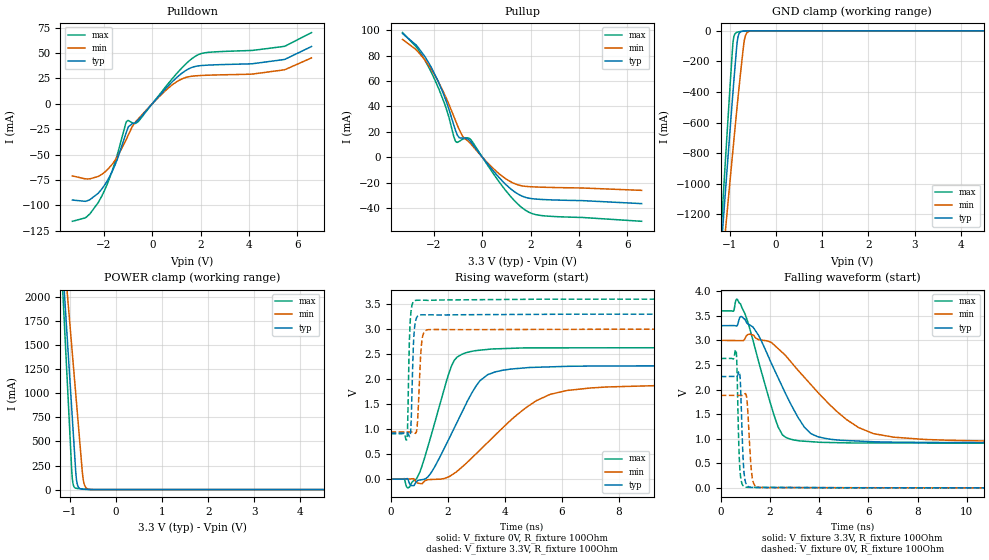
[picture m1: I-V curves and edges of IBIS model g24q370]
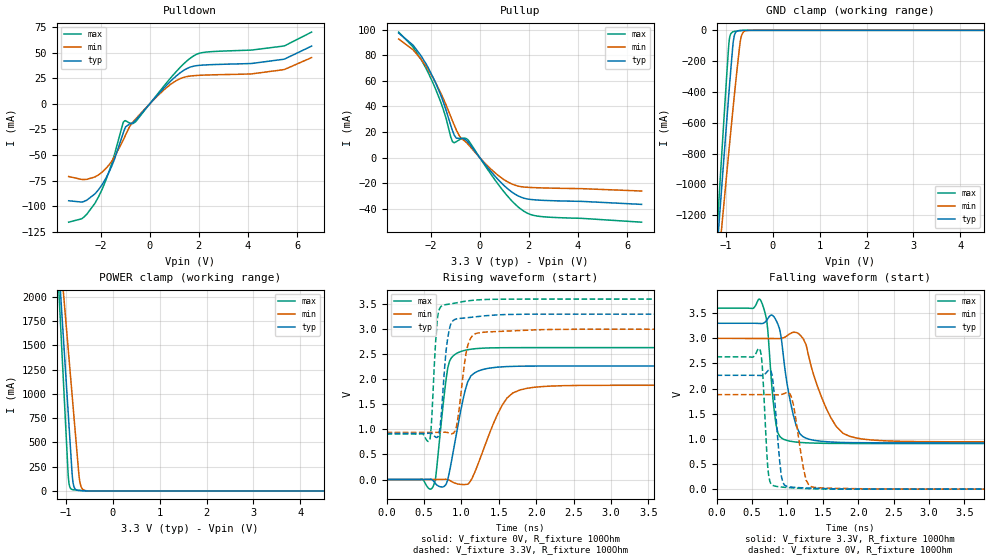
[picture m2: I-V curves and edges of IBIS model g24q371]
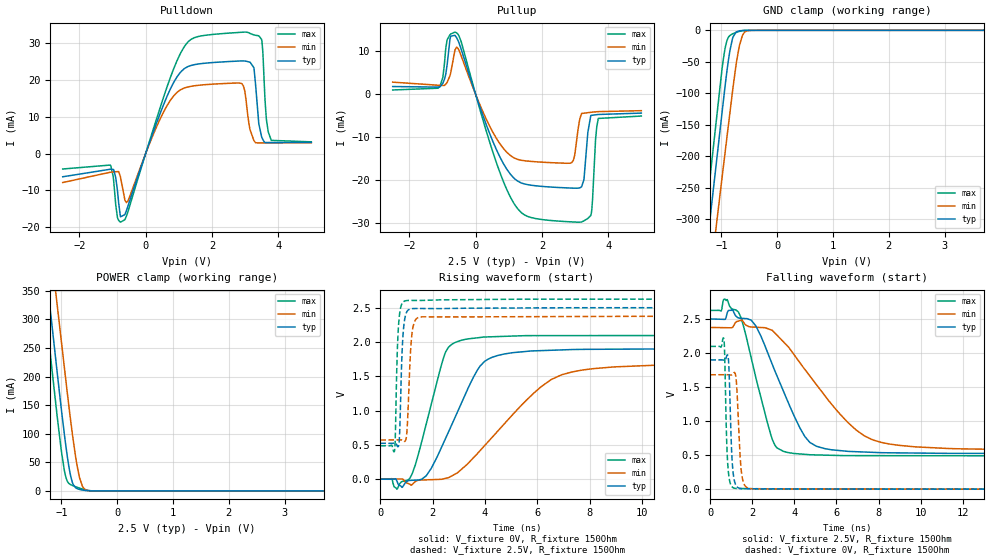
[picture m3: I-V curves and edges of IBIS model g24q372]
| Texas Instruments Incorporated
| Single Port 10/100 Mbps Eth Phys Layer Transceiver w/ Fiber Support
| Marketing part#   Voltage Range   Package-type   #pins/pkg drawing
| DP83620   2.375V - 3.6V   LLP   48-pin LLP
[IBIS Ver]   4.1
[Comment char]  |_char
[File name]   dp83620.ibs
[File Rev]   1.2
[Date]   11/01/2016
[Source]   Model built from spectre simulations at:
   Texas Instruments Incorporated.
   Analog-eLab, HPA
   12500 TI Blvd
   Dallas, TX -75243
   For Support e-mail: elab_ibis@list.ti.com
[Notes]   Revision History
   Rev 1.2: 11/1/2016
   - Update g24q370, g27q371 from DP83630
   Rev 1.1: 6/15/2016
   - New model for g24q37x buffer I/O at 2.5V operation.
   Rev 1.0: 05/2/2011
   -Pulldown & pullup non-monotonic for g24q37x modes reflect buffer behavior
   -osc25x1 POWER Clamp model stops at VCC. GND clamp shows 0 current at 0V.
   - C_comp although listed in numerical order of value are obtained from varying PVT conditions.
   For PVT conditions for each specific value, refer to the buffer description under respective [Model].
   IBIS model user is responsible for using appropriate C_comp to simulate for Signal Integrity.
[Disclaimer]  This model is designed as an aid for customers of Texas Instruments
 TI and its licensors and suppliers make no warranties, either expressed
 or implied, with respect to this  model, including the warranties of
 merchantability or fitness for a particular purpose.
 The model is provided solely on an "as is" basis. The entire risk as to
 its quality and performance is with the customer.
[Copyright] (C)Copyright 2016 Texas Instruments Incorporated.
   All rights reserved.
[Component]   DP83620
[Manufacturer]  Texas Instruments
[Package]
|   typ   min   max
R_pkg   0.359   0.180   0.442
L_pkg   2.373n   1.687n   2.945n
C_pkg   0.123p   0.108p   0.150p
[Pin]   signal_name   model_name   R_pin   L_pin   C_pin
1   TX_CLK   g24q37x   0.42936   2.873n   0.148196p
2   TX_EN   g24q37x   0.40013   2.628n   0.124306p
3   TXD_0   g24q37x   0.37267   2.418n   0.119907p
4   TXD_1   g24q37x   0.35187   2.266n   0.118634p
5   TXD_2   g24q37x   0.33473   2.147n   0.117883p
6   TXD_3   g24q37x   0.32586   2.085n   0.119334p
7   PWRDOWN/INTN   g24q37x   0.32558   2.084n   0.119406p
8   TCK   g24q37x   0.33356   2.137n   0.118268p
9   TDO   g24q37x   0.34873   2.244n   0.118339p
10   TMS   g24q37x   0.36988   2.399n   0.119828p
11   TRST#   g24q37x   0.39607   2.598n   0.123672p
12   TDI   g24q37x   0.42596   2.846n   0.146171p
13   RD-   NC   0.42552   2.846n   0.138036p
14   RD+   NC   0.39994   2.586n   0.114697p
15   CD_VSS   GND   0.21019   1.982n   0.12691p
16   TD-   NC   0.35238   2.219n   0.10829p
17   TD+   NC   0.33431   2.112n   0.109207p
18   ANAVSS   GND   0.18023   1.687n   0.130115p
19   ANA33VDD   POWER   0.32768   2.094n   0.114926p
20   VREF   NC   0.33377   2.159n   0.121083p
21   CLK_OUT_EN   g24q37x   0.34083   2.203n   0.118534p
22   PCF_EN   g24q37x   0.36206   2.35n   0.116057p
23   RESERVED   g24q37x   0.38591   2.551n   0.124689p
24   CLK_OUT   g24q37x   0.43535   2.929n   0.144582p
25   RESERVED   g24q37x   0.44243   2.945n   0.143157p
26   LED_ACT   g24q37x   0.40924   2.689n   0.124605p
27   LED_SPEED   g24q37x   0.38041   2.477n   0.121061p
28   LED_LINK   g24q37x   0.35858   2.311n   0.119803p
29   RESET_N   g24q37x   0.34101   2.179n   0.117093p
30   MDIO   g24q37x   0.32959   2.091n   0.115554p
31   MDC   g24q37x   0.32689   2.082n   0.117569p
32   IO_VDD   POWER   0.33388   2.126n   0.116848p
33   X2   osc25x2   0.35262   2.24n   0.115121p
34   X1   osc25x1   0.37844   2.403n   0.116058p
35   IO_CORE_VSS   GND   0.21929   2.112n   0.150154p
36   RESERVED   g24q37x   0.41951   2.799n   0.146508p
37   RESERVED   g24q37x   0.42645   2.861n   0.136214p
38   RX_CLK   g24q37x   0.40341   2.667n   0.120159p
39   RX_DV   g24q37x   0.37560   2.446n   0.114535p
40   CRS/CRS_DV   g24q37x   0.35301   2.276n   0.112899p
41   RX_ER   g24q37x   0.33596   2.154n   0.111927p
42   COL   g24q37x   0.32709   2.092n   0.111756p
43   RXD_3   g24q37x   0.32713   2.092n   0.11131p
44   RXD_2   g24q37x   0.33667   2.162n   0.112238p
45   RXD_1   g24q37x   0.35414   2.288n   0.113403p
46   RXD_0   g24q37x   0.37605   2.462n   0.117967p
47   IO_VSS   GND   0.39618   2.621n   0.122466p
48   IO_VDD   POWER   0.42506   2.862n   0.142308p
[Diff_pin]   inv_pin   vdiff   tdelay_typ   tdelay_min   tdelay_max
| The '+' pin is Diff_pin and the '-' pin is the inv_pin
14   13   0.100   0 0 0
17   16   0.100   0 0 0
[Model Selector]   g24q37x
g24q370   mode: SS = VSS, VDD = 3.3
g24q371   mode: SS = VDD, VDD = 3.3
g24q372   mode: SS = VSS, VDD = 2.5
g24q373   mode: SS = VDD, VDD = 2.5
| Models and submodels in the file (6): g24q370 (I/O), g24q371 (I/O), g24q372 (I/O), g24q373 (I/O), osc25x1 (Input), osc25x2 (Output)
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|   Model g24q370
[Model]   g24q370
Model_type   I/O
Polarity   Non-Inverting
Enable   Active-Low
Vinl = 0.8
Vinh = 2.0
Vmeas = 1.5
|   typ   min   max
C_comp   1.0640pF   1.0620pF   1.0670pF
[Voltage Range]   3.3   3   3.6
[Temperature Range]   25   125   -40
[Pullup Reference]   3.3   3   3.6
[Pulldown Reference]   0   0   0
[Power Clamp Reference]   3.3   3   3.6
[GND Clamp Reference]   0   0   0
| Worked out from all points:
|   slope of the pulldown table from 0 to 0.495 V, typ, clamps not added: 37.3 ohm
|   slope of the pullup table from 0 to 0.495 V, typ, clamps not added: 42.1 ohm
|   GND clamp passes 1 mA (typ) near -0.69 V on its own axis
|   POWER clamp passes 1 mA (typ) near -0.59 V on its own axis
|   falling waveform, V_fixture 3.3V, R_fixture 100Ohm: 20-80 % time 1.39ns typ, 2.41ns min, 911ps max; typ from 3.3 V to 0.919 V
|   rising waveform, V_fixture 0V, R_fixture 100Ohm: 20-80 % time 1.21ns typ, 2.18ns min, 795ps max; typ from 0 V to 2.27 V
|   rising waveform, V_fixture 3.3V, R_fixture 100Ohm: 20-80 % time 79.2ps typ, 104ps min, 68.6ps max; typ from 0.919 V to 3.3 V
|   falling waveform, V_fixture 0V, R_fixture 100Ohm: 20-80 % time 102ps typ, 134ps min, 86.2ps max; typ from 2.27 V to 0 V
[Pulldown]
|   Voltage   I(typ)   I(min)   I(max)
-3.3V     -94.78mA   -71.06mA   -115.7mA
-2.676V   -95.44mA   -74.02mA   -110.7mA
-2.092V   -84.17mA   -69.57mA   -91.23mA
-1.558V   -61.46mA   -56.42mA   -59.08mA
-1.073V   -28.13mA   -35.11mA   -17.82mA
-983.4mV  -22.58mA   -30.44mA   -16.52mA
-577.5mV  -16.03mA   -14.92mA   -17.52mA
838.2mV   21.93mA    18.83mA    24.99mA
1.62V     35.69mA    27.12mA    44.11mA
2.224V    38.02mA    28.13mA    50.44mA
5.452V    43.63mA    33.46mA    56.55mA
6.59V     56.49mA    45.27mA    70.2mA
[GND Clamp]
|   Voltage   I(typ)   I(min)   I(max)
-3.3V     -10.39A    -8.782A    -12.22A
-1.191V   -1.434A    -1.613A    -1.311A
-1.122V   -1.151A    -1.385A    -967.2mA
-1.102V   -1.07A     -1.32A     -869.6mA
-1.043V   -830.1mA   -1.127A    -579.2mA
-933.9mV  -400mA     -776mA     -77.86mA
-854.7mV  -108.3mA   -528mA     -9.646mA
-805.2mV  -20.45mA   -378.7mA   -6.059mA
-696.3mV  -1.135mA   -78.24mA   -2.129mA
-646.8mV  -417.3uA   -19.97mA   -1.017mA
-577.5mV  -93.99uA   -2.797mA   -240.5uA
6.59V     0A         0A         0A
[Pullup]
|   Voltage   I(typ)   I(min)   I(max)
-3.3V     97.33mA    92.68mA    98.1mA
-2.686V   87.17mA    83.6mA     85.57mA
-2.102V   70.37mA    68.84mA    66.51mA
-1.518V   45.28mA    47.6mA     39.67mA
-1.102V   20.69mA    28.41mA    12.28mA
-953.7mV  15.22mA    21.61mA    12.45mA
-825mV    15.02mA    16.78mA    13.99mA
-468.6mV  11.9mA     10.27mA    13.6mA
699.6mV   -16.19mA   -13.13mA   -19.54mA
1.67V     -30.88mA   -22.7mA    -40.23mA
2.501V    -33.35mA   -23.67mA   -46.09mA
6.59V     -36.58mA   -26.14mA   -50.5mA
[POWER Clamp]
|   Voltage   I(typ)   I(min)   I(max)
-3.3V     19.11A     15.19A     23.53A
-1.241V   2.989A     3.111A     2.924A
-963.6mV  899.3mA    1.533A     275.2mA
-953.7mV  824.7mA    1.477A     183.3mA
-933.9mV  675.5mA    1.365A     79.06mA
-874.5mV  227.9mA    1.027A     16.17mA
-854.7mV  111.6mA    914.3mA    13.23mA
-825mV    39.61mA    745.4mA    11.03mA
-716.1mV  3.952mA    138.9mA    6.502mA
-676.5mV  2.669mA    45.08mA    5.111mA
-597.3mV  1.12mA     4.928mA    2.691mA
6.59V     0A         0A         0A
[Ramp]
R_load = 100
|   typ   min   max
dV/dt_r   1.35904/1.20591e-09   1.12844/2.184e-09   1.57884/7.94904e-10
dV/dt_f   1.42833/1.38701e-09   1.2344/2.40837e-09   1.61561/9.11184e-10
[Falling Waveform]
V_fixture = 3.3V
V_fixture_min = 3V
V_fixture_max = 3.6V
R_fixture = 100Ohm
C_fixture = 0F
|   Time   V(typ)   V(min)   V(max)
0s        3.3V       3V         3.6V
519.7ps   3.301V     2.997V     3.592V
648.5ps   3.291V     2.996V     3.839V
807.3ps   3.483V     2.995V     3.741V
1.543ns   3.099V     3.014V     2.564V
2.336ns   2.237V     2.832V     1.237V
2.817ns   1.734V     2.584V     992.6mV
3.669ns   1.102V     2.098V     939.7mV
6.203ns   937.9mV    1.104V     913.2mV
15ns      919.5mV    942.7mV    907.3mV
[Rising Waveform]
V_fixture = 0V
V_fixture_min = 0V
V_fixture_max = 0V
R_fixture = 100Ohm
C_fixture = 0F
|   Time   V(typ)   V(min)   V(max)
0s        -4.136uV   4.39uV     1.746uV
609.7ps   -3.242mV   -188.8uV   -176.5mV
922.4ps   -45.19mV   -69.86mV   16.02mV
1.414ns   119.1mV    -9.452mV   856.1mV
2.134ns   904.1mV    76.49mV    2.258V
2.643ns   1.498V     309.3mV    2.527V
3.403ns   2.088V     729.1mV    2.594V
5.113ns   2.236V     1.567V     2.624V
6.203ns   2.255V     1.773V     2.625V
15ns      2.265V     1.881V     2.631V
[Rising Waveform]
V_fixture = 3.3V
V_fixture_min = 3V
V_fixture_max = 3.6V
R_fixture = 100Ohm
C_fixture = 0F
|   Time   V(typ)   V(min)   V(max)
0s        919.4mV    940.6mV    907.5mV
577.2ps   927.2mV    940.6mV    809.3mV
688ps     871.4mV    941.5mV    3.143V
722.6ps   1.164V     942.3mV    3.377V
801.9ps   2.691V     941.4mV    3.547V
858.3ps   3.102V     917mV      3.571V
947.7ps   3.26V      1.165V     3.578V
1.104ns   3.286V     2.789V     3.579V
1.289ns   3.286V     2.986V     3.575V
15ns      3.3V       3V         3.6V
[Falling Waveform]
|Gnd
V_fixture = 0V
V_fixture_min = 0V
V_fixture_max = 0V
R_fixture = 100Ohm
C_fixture = 0F
|   Time   V(typ)   V(min)   V(max)
0s        2.265V     1.881V     2.631V
621.6ps   2.26V      1.881V     2.803V
660.1ps   2.262V     1.881V     2.462V
779.1ps   2.302V     1.88V      376.9mV
915.1ps   545.8mV    1.881V     40.91mV
967.5ps   226.2mV    1.904V     21.05mV
1.079ns   42.12mV    1.727V     11.62mV
1.289ns   8.007mV    178.5mV    9.459mV
1.476ns   6.874mV    19.54mV    10.6mV
15ns      1.551uV    75.46uV    -1.284uV
|   Model g24q371
[Model]   g24q371
Model_type   I/O
Polarity   Non-Inverting
Enable   Active-Low
Vinl = 0.8
Vinh = 2.0
Vmeas = 1.5
|   typ   min   max
C_comp   1.0640pF   1.0620pF   1.0670pF
[Voltage Range]   3.3   3   3.6
[Temperature Range]   25   125   -40
[Pullup Reference]   3.3   3   3.6
[Pulldown Reference]   0   0   0
[Power Clamp Reference]   3.3   3   3.6
[GND Clamp Reference]   0   0   0
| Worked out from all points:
|   slope of the pulldown table from 0 to 0.495 V, typ, clamps not added: 37.3 ohm
|   slope of the pullup table from 0 to 0.495 V, typ, clamps not added: 42.1 ohm
|   GND clamp passes 1 mA (typ) near -0.69 V on its own axis
|   POWER clamp passes 1 mA (typ) near -0.59 V on its own axis
|   falling waveform, V_fixture 3.3V, R_fixture 100Ohm: 20-80 % time 170ps typ, 334ps min, 95.6ps max; typ from 3.3 V to 0.92 V
|   rising waveform, V_fixture 0V, R_fixture 100Ohm: 20-80 % time 179ps typ, 316ps min, 116ps max; typ from 0 V to 2.27 V
|   rising waveform, V_fixture 3.3V, R_fixture 100Ohm: 20-80 % time 82ps typ, 107ps min, 59.6ps max; typ from 0.92 V to 3.3 V
|   falling waveform, V_fixture 0V, R_fixture 100Ohm: 20-80 % time 80.8ps typ, 126ps min, 58.9ps max; typ from 2.27 V to 0 V
[Pulldown]
|   Voltage   I(typ)   I(min)   I(max)
-3.3V     -94.78mA   -71.06mA   -115.7mA
-2.676V   -95.44mA   -74.02mA   -110.7mA
-2.092V   -84.17mA   -69.57mA   -91.23mA
-1.558V   -61.46mA   -56.42mA   -59.08mA
-1.073V   -28.13mA   -35.11mA   -17.82mA
-983.4mV  -22.58mA   -30.44mA   -16.52mA
-577.5mV  -16.03mA   -14.92mA   -17.52mA
838.2mV   21.93mA    18.83mA    24.99mA
1.62V     35.69mA    27.12mA    44.11mA
2.224V    38.02mA    28.13mA    50.44mA
5.452V    43.63mA    33.46mA    56.55mA
6.59V     56.49mA    45.27mA    70.2mA
[GND Clamp]
|   Voltage   I(typ)   I(min)   I(max)
-3.3V     -10.39A    -8.782A    -12.22A
-1.191V   -1.434A    -1.613A    -1.311A
-1.122V   -1.151A    -1.385A    -967.2mA
-1.102V   -1.07A     -1.32A     -869.6mA
-1.043V   -830.1mA   -1.127A    -579.2mA
-933.9mV  -400mA     -776mA     -77.86mA
-854.7mV  -108.3mA   -528mA     -9.646mA
-805.2mV  -20.45mA   -378.7mA   -6.059mA
-696.3mV  -1.135mA   -78.24mA   -2.129mA
-646.8mV  -417.3uA   -19.97mA   -1.017mA
-577.5mV  -93.99uA   -2.797mA   -240.5uA
6.59V     0A         0A         0A
[Pullup]
|   Voltage   I(typ)   I(min)   I(max)
-3.3V     97.33mA    92.68mA    98.1mA
-2.686V   87.17mA    83.6mA     85.57mA
-2.102V   70.37mA    68.84mA    66.51mA
-1.518V   45.28mA    47.6mA     39.67mA
-1.102V   20.69mA    28.41mA    12.28mA
-953.7mV  15.22mA    21.61mA    12.45mA
-825mV    15.02mA    16.78mA    13.99mA
-468.6mV  11.9mA     10.27mA    13.6mA
699.6mV   -16.19mA   -13.13mA   -19.54mA
1.67V     -30.88mA   -22.7mA    -40.23mA
2.501V    -33.35mA   -23.67mA   -46.09mA
6.59V     -36.58mA   -26.14mA   -50.5mA
[POWER Clamp]
|   Voltage   I(typ)   I(min)   I(max)
-3.3V     19.11A     15.19A     23.53A
-1.241V   2.989A     3.111A     2.924A
-963.6mV  899.3mA    1.533A     275.2mA
-953.7mV  824.7mA    1.477A     183.3mA
-933.9mV  675.5mA    1.365A     79.06mA
-874.5mV  227.9mA    1.027A     16.17mA
-854.7mV  111.6mA    914.3mA    13.23mA
-825mV    39.61mA    745.4mA    11.03mA
-716.1mV  3.952mA    138.9mA    6.502mA
-676.5mV  2.669mA    45.08mA    5.111mA
-597.3mV  1.12mA     4.928mA    2.691mA
6.59V     0A         0A         0A
[Ramp]
R_load = 100
|   typ   min   max
dV/dt_r   1.35901/1.79012e-10   1.1284/3.1564e-10   1.57888/1.15789e-10
dV/dt_f   1.42826/1.69683e-10   1.23575/3.33638e-10   1.61558/9.55678e-11
[Falling Waveform]
V_fixture = 3.3V
V_fixture_min = 3V
V_fixture_max = 3.6V
R_fixture = 100Ohm
C_fixture = 0F
|   Time   V(typ)   V(min)   V(max)
0s        3.3V       3V         3.6V
619.5ps   3.296V     2.997V     3.765V
710.8ps   3.365V     2.997V     3.338V
798.2ps   3.449V     2.996V     1.778V
868ps     3.277V     2.996V     1.116V
1.102ns   1.383V     3.121V     940.4mV
1.266ns   1.014V     2.87V      922.3mV
1.688ns   933.9mV    1.253V     910.4mV
2.067ns   924.2mV    995.9mV    907.7mV
15ns      919.5mV    940.4mV    907.4mV
[Rising Waveform]
V_fixture = 0V
V_fixture_min = 0V
V_fixture_max = 0V
R_fixture = 100Ohm
C_fixture = 0F
|   Time   V(typ)   V(min)   V(max)
0s        -38.93uV   17.34uV    -47.63uV
619.5ps   -18.73mV   -74.43uV   -147.4mV
656.7ps   -83.05mV   -79.94uV   36.83mV
781.5ps   -122.4mV   4.755mV    1.821V
868ps     363.8mV    -37.69mV   2.43V
1.049ns   1.768V     -99.38mV   2.578V
1.19ns    2.138V     185mV      2.611V
1.611ns   2.253V     1.627V     2.63V
2.067ns   2.264V     1.853V     2.631V
15ns      2.265V     1.881V     2.631V
[Rising Waveform]
V_fixture = 3.3V
V_fixture_min = 3V
V_fixture_max = 3.6V
R_fixture = 100Ohm
C_fixture = 0F
|   Time   V(typ)   V(min)   V(max)
0s        919.5mV    940.4mV    907.4mV
570ps     924.6mV    940.5mV    767.2mV
596.4ps   922.5mV    940.5mV    1.026V
656.7ps   845.5mV    941mV      2.758V
696.4ps   886.2mV    941.9mV    3.358V
798.3ps   2.598V     942.1mV    3.49V
852.5ps   3.077V     918.3mV    3.502V
933.9ps   3.203V     1.057V     3.525V
1.102ns   3.232V     2.742V     3.567V
15ns      3.3V       3V         3.6V
[Falling Waveform]
|Gnd
V_fixture = 0V
V_fixture_min = 0V
V_fixture_max = 0V
R_fixture = 100Ohm
C_fixture = 0F
|   Time   V(typ)   V(min)   V(max)
0s        2.265V     1.881V     2.631V
607.1ps   2.262V     1.881V     2.793V
738.3ps   2.369V     1.881V     255mV
798.3ps   2.125V     1.88V      73.33mV
868ps     945.9mV    1.878V     50.02mV
958.1ps   84.16mV    1.904V     37.39mV
1.064ns   39.83mV    1.807V     26.57mV
1.266ns   23.97mV    179.9mV    12.15mV
1.399ns   16.58mV    32.99mV    6.609mV
15ns      39.27uV    17.32uV    47.44uV
|   Model g24q372
[Model]   g24q372
Model_type   I/O
Polarity   Non-Inverting
Vinl = 0.8000V
Vinh = 2.0000V
Vmeas = 1.25
Vref = 2.5
Cref = 15pF
Rref = 150
|   typ   min   max
|   (slow PVT)   (nom PVT)   (fast PVT)
C_comp   0.448p   0.445p   0.450p
|C_comp (ON state)   0.448p   0.445p   0.450p
|C_comp (OFF state)   0.441p   0.438p   0.444p
[Voltage Range]   2.5   2.375   2.625
[Temperature Range]   27   125   -40
[Pullup Reference]   2.5   2.375   2.625
[Pulldown Reference]   -0   -0   -0
[Power Clamp Reference]   2.5   2.375   2.625
[GND Clamp Reference]   0   0   0
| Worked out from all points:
|   slope of the pulldown table from 0 to 0.375 V, typ, clamps not added: 39.9 ohm
|   slope of the pullup table from 0 to 0.375 V, typ, clamps not added: 46 ohm
|   GND clamp passes 1 mA (typ) near -0.68 V on its own axis
|   POWER clamp passes 1 mA (typ) near -0.59 V on its own axis
|   falling waveform, V_fixture 2.5V, R_fixture 150Ohm: 20-80 % time 1.63ns typ, 2.82ns min, 1.03ns max; typ from 2.5 V to 0.523 V
|   rising waveform, V_fixture 0V, R_fixture 150Ohm: 20-80 % time 1.37ns typ, 2.52ns min, 852ps max; typ from 0 V to 1.9 V
|   rising waveform, V_fixture 2.5V, R_fixture 150Ohm: 20-80 % time 109ps typ, 131ps min, 98.5ps max; typ from 0.523 V to 2.5 V
|   falling waveform, V_fixture 0V, R_fixture 150Ohm: 20-80 % time 130ps typ, 169ps min, 114ps max; typ from 1.9 V to 0 V
[Pulldown]
|   Voltage   I(typ)   I(min)   I(max)
-2.5V     -6.301mA   -7.87mA    -4.193mA
-1.067V   -4.261mA   -5.073mA   -3.123mA
-850mV    -10.03mA   -4.9mA     -17.38mA
-625mV    -16.56mA   -12.65mA   -17.93mA
957.5mV   20.95mA    16.67mA    25.42mA
1.895V    24.59mA    18.74mA    32.18mA
2.9V      25.12mA    18.92mA    32.89mA
3.147V    24.76mA    6.409mA    32.57mA
3.268V    22.92mA    3.458mA    32.16mA
3.41V     8.064mA    2.886mA    31.93mA
3.785V    2.989mA    2.887mA    3.573mA
4.992V    2.997mA    2.896mA    3.167mA
[GND Clamp]
|   Voltage   I(typ)   I(min)   I(max)
-2.5V     -1.339A    -1.384A    -1.315A
-1.66V    -661.3mA   -738.1mA   -610.7mA
-1.278V   -357.2mA   -448.8mA   -294.4mA
-1.21V    -303.9mA   -398.2mA   -238.9mA
-1.165V   -268.5mA   -364.6mA   -202mA
-992.5mV  -133.4mA   -236.7mA   -63.79mA
-940mV    -92.71mA   -198.1mA   -31.44mA
-850mV    -33.15mA   -132.4mA   -8.308mA
-730mV    -2.402mA   -50.04mA   -3.042mA
-625mV    -273.8uA   -8.504mA   -672.2uA
-497.5mV  -14.45uA   -281.2uA   -27.02uA
4.992V    0A         0A         0A
[Pullup]
|   Voltage   I(typ)   I(min)   I(max)
-2.5V     1.836mA    2.857mA    1.034mA
-1.127V   1.702mA    2.137mA    1.448mA
-857.5mV  7.029mA    2.836mA    12.75mA
-752.5mV  13.55mA    4.976mA    14.05mA
-572.5mV  13.18mA    11.02mA    14.33mA
950mV     -17.53mA   -13.54mA   -22.34mA
2.105V    -21.46mA   -15.81mA   -29.2mA
2.9V      -21.79mA   -15.83mA   -29.65mA
3.192V    -21.49mA   -4.43mA    -29.66mA
3.47V     -4.893mA   -4.159mA   -28.16mA
3.695V    -4.663mA   -3.998mA   -5.585mA
4.992V    -4.342mA   -3.781mA   -5.028mA
[POWER Clamp]
|   Voltage   I(typ)   I(min)   I(max)
-2.5V     1.468A     1.541A     1.422A
-1.165V   285.5mA    400.7mA    208.4mA
-1.157V   278.9mA    394.3mA    201.6mA
-1.075V   206.1mA    324.2mA    129.3mA
-992.5mV  135.3mA    254mA      63.99mA
-932.5mV  87.45mA    203mA      28.56mA
-835mV    26.06mA    123.1mA    10.98mA
-790mV    11.35mA    89.4mA     9.001mA
-722.5mV  4.146mA    45.6mA     6.498mA
-625mV    1.561mA    8.387mA    3.375mA
-490mV    160.1uA    282.6uA    541.7uA
4.992V    0A         0A         0A
[Ramp]
R_load = 150
|   typ   min   max
dV/dt_r   1.13883/1.36699e-09   1.00801/2.51562e-09   1.25786/8.51473e-10
dV/dt_f   1.18607/1.62971e-09   1.0815/2.81583e-09   1.28244/1.02914e-09
[Falling Waveform]
V_fixture = 2.5V
V_fixture_min = 2.375V
V_fixture_max = 2.625V
R_fixture = 150Ohm
C_fixture = 0F
|   Time   V(typ)   V(min)   V(max)
0s        2.5V       2.375V     2.625V
514.9ps   2.495V     2.372V     2.616V
685.2ps   2.493V     2.371V     2.792V
1.338ns   2.515V     2.469V     2.602V
2.175ns   2.394V     2.378V     1.628V
2.885ns   1.882V     2.34V      791.5mV
3.479ns   1.438V     2.164V     555.1mV
4.732ns   686.6mV    1.663V     505.7mV
7.727ns   540.6mV    723.5mV    492.2mV
19.9ns    523.2mV    572.5mV    487.6mV
[Rising Waveform]
V_fixture = 0V
V_fixture_min = 0V
V_fixture_max = 0V
R_fixture = 150Ohm
C_fixture = 0F
|   Time   V(typ)   V(min)   V(max)
0s        567.5pV    22.84nV    158pV
632.7ps   -25.38mV   3.156mV    -144.7mV
1.132ns   -16.86mV   -73.32mV   15.86mV
1.753ns   49.26mV    -9.286mV   800.5mV
2.447ns   555.2mV    8.662mV    1.804V
3.082ns   1.094V     138.1mV    2.023V
4.109ns   1.747V     541.5mV    2.074V
6.127ns   1.874V     1.343V     2.092V
7.327ns   1.89V      1.563V     2.093V
19.9ns    1.898V     1.68V      2.096V
[Rising Waveform]
V_fixture = 2.5V
V_fixture_min = 2.375V
V_fixture_max = 2.625V
R_fixture = 150Ohm
C_fixture = 0F
|   Time   V(typ)   V(min)   V(max)
0s        523.2mV    571.3mV    487.6mV
555.5ps   527.6mV    573mV      439.3mV
645.5ps   487mV      573.3mV    1.81V
702.2ps   489.4mV    573.5mV    2.266V
850.1ps   1.991V     571.1mV    2.571V
953.1ps   2.371V     556.3mV    2.599V
1.018ns   2.443V     693.3mV    2.603V
1.211ns   2.485V     2.12V      2.605V
1.511ns   2.487V     2.363V     2.605V
19.9ns    2.5V       2.375V     2.625V
[Falling Waveform]
|Gnd
V_fixture = 0V
V_fixture_min = 0V
V_fixture_max = 0V
R_fixture = 150Ohm
C_fixture = 0F
|   Time   V(typ)   V(min)   V(max)
0s        1.898V     1.68V      2.096V
645.5ps   1.894V     1.68V      2.207V
779.5ps   1.954V     1.68V      705.2mV
850.1ps   1.944V     1.68V      287.1mV
1.016ns   546.8mV    1.678V     41.67mV
1.132ns   146.3mV    1.712V     14.9mV
1.238ns   47.12mV    1.586V     10.19mV
1.464ns   8.117mV    294mV      8.927mV
1.825ns   5.652mV    12.58mV    8.505mV
19.9ns    4.163uV    30.86uV    -5.271uV
